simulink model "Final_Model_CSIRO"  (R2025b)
settings: Solver=ode23tb  StartTime=0.0  StopTime=50  RelTol=1e-3
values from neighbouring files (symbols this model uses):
  C_4 = 0.1670*C_b    (= 1.00487241952e-06)    [VSM_CSIRO.m]    (also in VSM.m)
  C_6 = 0.2835*C_b    (= 1.70587623314e-06)    [VSM_CSIRO.m]    (also in VSM.m)
  C_8 = 0.2275*C_b    (= 1.36891302659e-06)    [VSM_CSIRO.m]    (also in VSM.m)
  C_dc = 0.008*(n)    (= 1.6)    [VSM_CSIRO.m]    (also in VSM.m)
  C_f = n*300*10^-6    (= 0.06)    [VSM_CSIRO.m]    (also in VSM.m)
  D_p = (1/(m_p*w_b))    (= 101321.183642)    [VSM_CSIRO.m]    (also in VSM.m)
  droop_percentage = 1    [VSM_CSIRO.m]    (also in VSM.m = 5)
  i_ll = -1.15*(S_b/Vdc_n)-i_loss_dc    [VSM_CSIRO.m]    (also in VSM.m)
  i_ul = 1.15*(S_b/Vdc_n)+i_loss_dc    [VSM_CSIRO.m]    (also in VSM.m)
  J = D_p*tau_f    (= 2026.42367285)    [VSM_CSIRO.m]    (also in VSM.m)
  k_dc = eta_1/(Vdc_n*m_p)    [VSM_CSIRO.m]    (also in VSM.m)
  K_p = (1/Vdc_n)    [VSM_CSIRO.m]    (also in VSM.m)
  K_r = 1/R_dc    [VSM_CSIRO.m]    (also in VSM.m)
  Kff_i = 1    [VSM_CSIRO.m]    (also in VSM.m)
  Kff_v = 1    [VSM_CSIRO.m]    (also in VSM.m)
  Ki_i = (1/n)*1.19    (= 0.00595)    [VSM_CSIRO.m]    (also in VSM.m)
  Ki_v = (n)*1.161022    (= 232.2044)    [VSM_CSIRO.m]    (also in VSM.m)
  ki_v_ac = 4*5.2500e-04    (= 0.0021)    [VSM_CSIRO.m]    (also in VSM.m)
  Kp_i = 0.738891    [VSM_CSIRO.m]    (also in VSM.m)
  Kp_v = 0.52    [VSM_CSIRO.m]    (also in VSM.m)
  kp_v_ac = 0.001    [VSM_CSIRO.m]    (also in VSM.m)
  L1_pu = 1*0.0186/m    (= 0.000186)    [VSM_CSIRO.m]    (also in VSM.m)
  L_45 = L_lines(2)    [VSM_CSIRO.m]    (also in VSM.m)
  L_56 = L_lines(3)    [VSM_CSIRO.m]    (also in VSM.m)
  L_67 = L_lines(5)    [VSM_CSIRO.m]    (also in VSM.m)
  L_78 = L_lines(6)    [VSM_CSIRO.m]    (also in VSM.m)
  L_89 = L_lines(8)    [VSM_CSIRO.m]    (also in VSM.m)
  L_94 = L_lines(9)    [VSM_CSIRO.m]    (also in VSM.m)
  L_f = (1/n)*200*10^-6    (= 1e-06)    [VSM_CSIRO.m]    (also in VSM.m)
  n = 200    [VSM_CSIRO.m]    (also in VSM.m)
  pl = S_b*ps    (= 75000000)    [VSM_CSIRO.m]    (also in VSM.m)
  ps = base/3    (= 0.75)    [VSM_CSIRO.m]    (also in VSM.m)
  R1_pu = 1*0.00734/m    (= 7.34e-05)    [VSM_CSIRO.m]    (also in VSM.m)
  R_45 = R_lines(2)    [VSM_CSIRO.m]    (also in VSM.m)
  R_56 = R_lines(3)    [VSM_CSIRO.m]    (also in VSM.m)
  R_67 = R_lines(5)    [VSM_CSIRO.m]    (also in VSM.m)
  R_78 = R_lines(6)    [VSM_CSIRO.m]    (also in VSM.m)
  R_89 = R_lines(8)    [VSM_CSIRO.m]    (also in VSM.m)
  R_94 = R_lines(9)    [VSM_CSIRO.m]    (also in VSM.m)
  R_dc = (Vdc_n/(0.05*(S_b)/Vdc_n))    [VSM_CSIRO.m]    (also in VSM.m)
  R_f = 0.001/n    (= 5e-06)    [VSM_CSIRO.m]    (also in VSM.m)
  S_b = 100*(10^6)    (= 100000000)    [VSM_CSIRO.m]    (also in VSM.m)
  S_bt = S_b    (= 100000000)    [VSM_CSIRO.m]    (also in VSM.m)
  T_en = T_load-0.5    (= 44.5)    [VSM_CSIRO.m]    (also in VSM.m = 24.5)
  t_l = 2    [VSM_CSIRO.m]
  tau_dc = 0.05    [VSM_CSIRO.m]    (also in VSM.m)
  tau_g = 5    [VSM_CSIRO.m]    (also in VSM.m)
  V1_rms = 1000    [VSM_CSIRO.m]    (also in VSM.m)
  V2_rms = 13800    [VSM_CSIRO.m]    (also in VSM.m)
  V_m = sqrt(2/3)*V1_rms    [VSM_CSIRO.m]    (also in VSM.m)
  Vdc_n = 3*V_m    [VSM_CSIRO.m]    (also in VSM.m)
  w_b = 2*pi*f_b    (= 314.159265359)    [VSM_CSIRO.m]    (also in VSM.m)
  w_f = 2*pi*5    (= 31.4159265359)    [VSM_CSIRO.m]    (also in VSM.m)
undefined symbols (not defined in the file or in its folder): D1, Delta, DiscIntNeverNeededParam, i_dc
libraries: spsSeriesRLCBranchLib x142, spsThreePhaseVIMeasurementLib x69, slpidlib x44, spsabctodq0Lib x44, spsVoltageMeasurementLib x28, spsGroundLib x23, spsThreePhaseBreakerLib x23, spsThreePhaseParallelRLCLoadLib x21, spsdq0toabcLib x16, spsUniversalBridgeLib x16, spsPowerPositiveSequenceLib x14, spsDCVoltageSourceLib x14
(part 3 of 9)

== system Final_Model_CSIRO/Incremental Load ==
  Base Load {1..6,8..12} (11 alike) : spsThreePhaseParallelRLCLoadLib/Three-Phase Parallel RLC Load  LConnTagsString=A|B|C  Configuration=Y (grounded)  NominalVoltage=230e3  Vabc=[1e3 1e3 1e3]  Vabcp=[1e3 1e3 1e3]  NominalFrequency=50  UnbalancedPower=off  ActivePower=pl-pl+10.04e6  InductivePower=0  CapacitivePower=0  Pabc=[10e3 9e3 11e3]  QLabc=[100 90 110]  QCabc=[100 90 110]  Pabcp=[10e3 9e3 11e3]  QLabcp=[100 90 110]  QCabcp=[100 90 110]  Measurements=None  LoadType=constant Z
  Base Load {7,13..18} (7 alike) : spsThreePhaseParallelRLCLoadLib/Three-Phase Parallel RLC Load  LConnTagsString=A|B|C  Configuration=Y (grounded)  NominalVoltage=230e3  Vabc=[1e3 1e3 1e3]  Vabcp=[1e3 1e3 1e3]  NominalFrequency=50  UnbalancedPower=off  ActivePower=pl-pl+10e6  InductivePower=0  CapacitivePower=0  Pabc=[10e3 9e3 11e3]  QLabc=[100 90 110]  QCabc=[100 90 110]  Pabcp=[10e3 9e3 11e3]  QLabcp=[100 90 110]  QCabcp=[100 90 110]  Measurements=None  LoadType=constant Z
  Three-Phase Breaker1 : spsThreePhaseBreakerLib/Three-Phase Breaker  InitialState=open  SwitchA=on  SwitchB=on  SwitchC=on  SwitchTimes=10+2*t_l  External=off  BreakerResistance=0.01  SnubberResistance=1e6  SnubberCapacitance=inf  Measurements=None
  Three-Phase Breaker10 : spsThreePhaseBreakerLib/Three-Phase Breaker  InitialState=open  SwitchA=on  SwitchB=on  SwitchC=on  SwitchTimes=10+9*t_l  External=off  BreakerResistance=0.01  SnubberResistance=1e6  SnubberCapacitance=inf  Measurements=None
  Three-Phase Breaker11 : spsThreePhaseBreakerLib/Three-Phase Breaker  InitialState=open  SwitchA=on  SwitchB=on  SwitchC=on  SwitchTimes=10+10*t_l  External=off  BreakerResistance=0.01  SnubberResistance=1e6  SnubberCapacitance=inf  Measurements=None
  Three-Phase Breaker12 : spsThreePhaseBreakerLib/Three-Phase Breaker  InitialState=open  SwitchA=on  SwitchB=on  SwitchC=on  SwitchTimes=10+11*t_l  External=off  BreakerResistance=0.01  SnubberResistance=1e6  SnubberCapacitance=inf  Measurements=None
  Three-Phase Breaker13 : spsThreePhaseBreakerLib/Three-Phase Breaker  InitialState=open  SwitchA=on  SwitchB=on  SwitchC=on  SwitchTimes=10+15*t_l  External=off  BreakerResistance=0.01  SnubberResistance=1e6  SnubberCapacitance=inf  Measurements=None
  Three-Phase Breaker14 : spsThreePhaseBreakerLib/Three-Phase Breaker  InitialState=open  SwitchA=on  SwitchB=on  SwitchC=on  SwitchTimes=10+16*t_l  External=off  BreakerResistance=0.01  SnubberResistance=1e6  SnubberCapacitance=inf  Measurements=None
  Three-Phase Breaker15 : spsThreePhaseBreakerLib/Three-Phase Breaker  InitialState=open  SwitchA=on  SwitchB=on  SwitchC=on  SwitchTimes=10+17*t_l  External=off  BreakerResistance=0.01  SnubberResistance=1e6  SnubberCapacitance=inf  Measurements=None
  Three-Phase Breaker16 : spsThreePhaseBreakerLib/Three-Phase Breaker  InitialState=open  SwitchA=on  SwitchB=on  SwitchC=on  SwitchTimes=10+12*t_l  External=off  BreakerResistance=0.01  SnubberResistance=1e6  SnubberCapacitance=inf  Measurements=None
  Three-Phase Breaker17 : spsThreePhaseBreakerLib/Three-Phase Breaker  InitialState=open  SwitchA=on  SwitchB=on  SwitchC=on  SwitchTimes=10+13*t_l  External=off  BreakerResistance=0.01  SnubberResistance=1e6  SnubberCapacitance=inf  Measurements=None
  Three-Phase Breaker18 : spsThreePhaseBreakerLib/Three-Phase Breaker  InitialState=open  SwitchA=on  SwitchB=on  SwitchC=on  SwitchTimes=10+14*t_l  External=off  BreakerResistance=0.01  SnubberResistance=1e6  SnubberCapacitance=inf  Measurements=None
  Three-Phase Breaker2 : spsThreePhaseBreakerLib/Three-Phase Breaker  InitialState=open  SwitchA=on  SwitchB=on  SwitchC=on  SwitchTimes=10+t_l  External=off  BreakerResistance=0.01  SnubberResistance=1e6  SnubberCapacitance=inf  Measurements=None
  Three-Phase Breaker3 : spsThreePhaseBreakerLib/Three-Phase Breaker  InitialState=open  SwitchA=on  SwitchB=on  SwitchC=on  SwitchTimes=10  External=off  BreakerResistance=0.01  SnubberResistance=1e6  SnubberCapacitance=inf  Measurements=None
  Three-Phase Breaker4 : spsThreePhaseBreakerLib/Three-Phase Breaker  InitialState=open  SwitchA=on  SwitchB=on  SwitchC=on  SwitchTimes=10+3*t_l  External=off  BreakerResistance=0.01  SnubberResistance=1e6  SnubberCapacitance=inf  Measurements=None
  Three-Phase Breaker5 : spsThreePhaseBreakerLib/Three-Phase Breaker  InitialState=open  SwitchA=on  SwitchB=on  SwitchC=on  SwitchTimes=10+4*t_l  External=off  BreakerResistance=0.01  SnubberResistance=1e6  SnubberCapacitance=inf  Measurements=None
  Three-Phase Breaker6 : spsThreePhaseBreakerLib/Three-Phase Breaker  InitialState=open  SwitchA=on  SwitchB=on  SwitchC=on  SwitchTimes=10+5*t_l  External=off  BreakerResistance=0.01  SnubberResistance=1e6  SnubberCapacitance=inf  Measurements=None
  Three-Phase Breaker7 : spsThreePhaseBreakerLib/Three-Phase Breaker  InitialState=open  SwitchA=on  SwitchB=on  SwitchC=on  SwitchTimes=10+6*t_l  External=off  BreakerResistance=0.01  SnubberResistance=1e6  SnubberCapacitance=inf  Measurements=None
  Three-Phase Breaker8 : spsThreePhaseBreakerLib/Three-Phase Breaker  InitialState=open  SwitchA=on  SwitchB=on  SwitchC=on  SwitchTimes=10+7*t_l  External=off  BreakerResistance=0.01  SnubberResistance=1e6  SnubberCapacitance=inf  Measurements=None
  Three-Phase Breaker9 : spsThreePhaseBreakerLib/Three-Phase Breaker  InitialState=open  SwitchA=on  SwitchB=on  SwitchC=on  SwitchTimes=10+8*t_l  External=off  BreakerResistance=0.01  SnubberResistance=1e6  SnubberCapacitance=inf  Measurements=None
  C : PMIOPort  Side=Left
  B : PMIOPort  Port=2  Side=Left
  A : PMIOPort  Port=3  Side=Left
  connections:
  Three-Phase Breaker10/LConn2 -- Three-Phase Breaker11/LConn2 -- Three-Phase Breaker9/LConn2 -- Three-Phase Breaker8/LConn2 -- Three-Phase Breaker3/LConn2 -- B/RConn1 -- Three-Phase Breaker2/LConn2 -- Three-Phase Breaker1/LConn2 -- Three-Phase Breaker4/LConn2 -- Three-Phase Breaker5/LConn2 -- Three-Phase Breaker6/LConn2 -- Three-Phase Breaker7/LConn2
  Three-Phase Breaker2/RConn3 -- Base Load 1/LConn1
  Three-Phase Breaker10/LConn1 -- Three-Phase Breaker11/LConn1 -- Three-Phase Breaker9/LConn1 -- Three-Phase Breaker8/LConn1 -- Three-Phase Breaker7/LConn1 -- Three-Phase Breaker2/LConn1 -- A/RConn1 -- Three-Phase Breaker3/LConn1 -- Three-Phase Breaker1/LConn1 -- Three-Phase Breaker4/LConn1 -- Three-Phase Breaker5/LConn1 -- Three-Phase Breaker6/LConn1
  Three-Phase Breaker3/RConn1 -- Base Load 7/LConn3
  Three-Phase Breaker10/LConn3 -- Three-Phase Breaker11/LConn3 -- Three-Phase Breaker9/LConn3 -- Three-Phase Breaker8/LConn3 -- Three-Phase Breaker3/LConn3 -- C/RConn1 -- Three-Phase Breaker2/LConn3 -- Three-Phase Breaker1/LConn3 -- Three-Phase Breaker4/LConn3 -- Three-Phase Breaker5/LConn3 -- Three-Phase Breaker6/LConn3 -- Three-Phase Breaker7/LConn3
  Three-Phase Breaker2/RConn1 -- Base Load 1/LConn3
  Three-Phase Breaker3/RConn2 -- Base Load 7/LConn2
  Three-Phase Breaker3/RConn3 -- Base Load 7/LConn1
  Three-Phase Breaker2/RConn2 -- Base Load 1/LConn2
  Three-Phase Breaker1/RConn1 -- Base Load 2/LConn3
  Three-Phase Breaker1/RConn2 -- Base Load 2/LConn2
  Three-Phase Breaker4/RConn1 -- Base Load 3/LConn3
  Three-Phase Breaker4/RConn2 -- Base Load 3/LConn2
  Three-Phase Breaker5/RConn1 -- Base Load 4/LConn3
  Three-Phase Breaker5/RConn2 -- Base Load 4/LConn2
  Three-Phase Breaker1/RConn3 -- Base Load 2/LConn1
  Three-Phase Breaker4/RConn3 -- Base Load 3/LConn1
  Three-Phase Breaker6/RConn2 -- Base Load 5/LConn2
  Three-Phase Breaker6/RConn1 -- Base Load 5/LConn3
  Three-Phase Breaker5/RConn3 -- Base Load 4/LConn1
  Three-Phase Breaker6/RConn3 -- Base Load 5/LConn1
  Three-Phase Breaker7/RConn2 -- Base Load 6/LConn2
  Three-Phase Breaker7/RConn1 -- Base Load 6/LConn3
  Three-Phase Breaker7/RConn3 -- Base Load 6/LConn1
  Three-Phase Breaker8/RConn1 -- Base Load 8/LConn3
  Three-Phase Breaker9/RConn1 -- Base Load 9/LConn3
  Three-Phase Breaker9/RConn3 -- Base Load 9/LConn1
  Three-Phase Breaker11/RConn2 -- Base Load 11/LConn2
  Three-Phase Breaker10/RConn3 -- Base Load 10/LConn1
  Three-Phase Breaker11/RConn1 -- Base Load 11/LConn3
  Three-Phase Breaker8/RConn3 -- Base Load 8/LConn1
  Three-Phase Breaker11/RConn3 -- Base Load 11/LConn1
  Three-Phase Breaker10/RConn2 -- Base Load 10/LConn2
  Three-Phase Breaker12/RConn1 -- Base Load 12/LConn3
  Three-Phase Breaker8/RConn2 -- Base Load 8/LConn2
  Three-Phase Breaker10/RConn1 -- Base Load 10/LConn3
  Three-Phase Breaker12/RConn2 -- Base Load 12/LConn2
  Three-Phase Breaker9/RConn2 -- Base Load 9/LConn2
  Three-Phase Breaker14/RConn3 -- Base Load 14/LConn1
  Three-Phase Breaker16/RConn2 -- Base Load 16/LConn2
  Three-Phase Breaker16/RConn3 -- Base Load 16/LConn1
  Three-Phase Breaker17/RConn3 -- Base Load 17/LConn1
  Three-Phase Breaker17/RConn2 -- Base Load 17/LConn2
  Three-Phase Breaker13/RConn2 -- Base Load 13/LConn2
  Three-Phase Breaker15/RConn2 -- Base Load 15/LConn2
  Three-Phase Breaker13/RConn3 -- Base Load 13/LConn1
  Three-Phase Breaker18/RConn2 -- Base Load 18/LConn2
  Three-Phase Breaker18/RConn1 -- Base Load 18/LConn3
  Three-Phase Breaker14/RConn1 -- Base Load 14/LConn3
  Three-Phase Breaker14/RConn2 -- Base Load 14/LConn2
  Three-Phase Breaker17/RConn1 -- Base Load 17/LConn3
  Three-Phase Breaker15/RConn1 -- Base Load 15/LConn3
  Three-Phase Breaker15/RConn3 -- Base Load 15/LConn1
  Three-Phase Breaker18/RConn3 -- Base Load 18/LConn1
  Three-Phase Breaker13/RConn1 -- Base Load 13/LConn3
  Three-Phase Breaker16/RConn1 -- Base Load 16/LConn3
  Three-Phase Breaker18/LConn2 -- Three-Phase Breaker15/LConn2 -- Three-Phase Breaker14/LConn2 -- Three-Phase Breaker13/LConn2
  Three-Phase Breaker15/LConn1 -- Three-Phase Breaker14/LConn1 -- Three-Phase Breaker18/LConn1 -- Three-Phase Breaker13/LConn1
  Three-Phase Breaker15/LConn3 -- Three-Phase Breaker14/LConn3 -- Three-Phase Breaker18/LConn3 -- Three-Phase Breaker13/LConn3
  Base Load 12/LConn1 -- Three-Phase Breaker12/RConn3
  Three-Phase Breaker12/LConn2 -- Three-Phase Breaker16/LConn2
  Three-Phase Breaker12/LConn1 -- Three-Phase Breaker16/LConn1
  Three-Phase Breaker12/LConn3 -- Three-Phase Breaker16/LConn3

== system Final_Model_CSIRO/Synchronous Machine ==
  Pset : Inport
  Bus Selector3 : BusSelector  OutputSignals="dq0 components.Stator voltage  vq (pu),dq0 components.Stator voltage  vd (pu),Output active power   Peo (pu),Output reactive power  Qeo (pu),Mechanical.Rotor mechanical angle  theta (deg),Mechanical.Rotor speed deviation  dw (pu),dq0 components.Field current  ifd (pu),Mechanical.Rotor speed  wm (pu)"
  Gain : Gain  Gain=50
  Generic Power System Stabilizer : spsGenericPowerSystemStabilizerLib/Generic Power System Stabilizer  Tsensor=30e-4  K=2.5  Twashout=2  Tleadlag1=[2*50e-3 0.01*20e-3]  Tleadlag2=[2*3 0.1*5.4]  VSlimits=2*[-0.15 0.15]  Vinit=0  Plot_On=off  MagdB_On=on  FreqRange=logspace(-2,2,500)
  LTI System3 : cstblocks/LTI System  sys=tf(1,[tau_g 1])  IC=[]  PadeOrder=0
  Mux1 : Mux  Inputs=2
  Mux3 : Mux  Inputs=2
  Positive Sequence Voltage1 : Fcn  Expr=sqrt(u(1)^2 + u(2)^2)
  Positive Sequence Voltage2 : Fcn  Expr=sqrt(u(1)^2 + u(2)^2)
  ST1A Excitation System : spsST1AExcitationSystemLib/ST1A Excitation System  Tr=20e-4  KaTa=[210 0.001]  VIminmax=[-999 +999]  VAminmax=[-999 999]  VRminmax=[-6.0 6.43]  KfTf=[0.001 1]  TbTc=[0 0 0 0]  KLR=1  ILR=2  Kc=0.038  v0=[1 1]  TsBlock=0
  Subsystem2 : Subsystem
  Synchronous Machine pu Fundamental : spsSynchronousMachinepuFundamentalLib/Synchronous Machine pu Fundamental  PresetModel=No  MechanicalLoad=Mechanical power Pm  ShowDetailedParameters=on  RotorType=Salient-pole  Units=per unit fundamental parameters  MeasurementBus=off  NominalParameters="[100E6  V2_rms   50]"  Stator="[ 2.85E-03  0.114  1.19  0.36 ]"  Field="[ 5.79E-04  0.114]"  Dampers2=[0.0652, 0.5134, 0.0287, 0.2553, 7.765e-3, 0.9167 ]  Dampers1="[ 1.17E-02  0.182  1.97E-02  0.384 ]"  Mechanical=[ 3.7 0 20]  PolePairs=20  InitialConditions="[ 0  0  0  0  0  0  0  0  1 ]"  SetSaturation=off  Saturation=[0.6404,0.7127,0.8441,0.9214,0.9956,1.082,1.19,1.316,1.457;0.7,0.7698,0.8872,0.9466,0.9969,1.046,1.1,1.151,1.201]  LoadFlowParameters=[1,0,0,0,0]  TsPowergui=0  TsBlock=-1  IterativeModel=Trapezoidal non iterative  IterativeDiscreteModel=Trapezoidal non iterative  BusType=PV  Pref=0  Qref=0  Qmin=-inf  Qmax=inf  PLF=0  QLF=0
  Terminal Load : spsThreePhaseParallelRLCLoadLib/Three-Phase Parallel RLC Load  LConnTagsString=A|B|C  Configuration=Y (grounded)  NominalVoltage=V2_rms  Vabc=[1e3 1e3 1e3]  Vabcp=[1e3 1e3 1e3]  NominalFrequency=50  UnbalancedPower=off  ActivePower=1  InductivePower=0  CapacitivePower=0  Pabc=[10e3 9e3 11e3]  QLabc=[100 90 110]  QCabc=[100 90 110]  Pabcp=[10e3 9e3 11e3]  QLabcp=[100 90 110]  QCabcp=[100 90 110]  Measurements=None  LoadType=constant Z
  wref6 : Constant
  wref7 : Constant
  A : PMIOPort  Side=Right
  B : PMIOPort  Port=2  Side=Right
  C : PMIOPort  Port=3  Side=Right
  f : Outport  VectorParamsAs1DForOutWhenUnconnected=off
  V : Outport  Port=2  VectorParamsAs1DForOutWhenUnconnected=off
  P : Outport  Port=3  VectorParamsAs1DForOutWhenUnconnected=off
  Theta : Outport  Port=4  VectorParamsAs1DForOutWhenUnconnected=off
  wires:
  Gain/1 -> f/1
  Pset/1 -> Subsystem2/1(P_ref)
  Positive Sequence Voltage2/1 -> V/1
  wref7/1 -> Subsystem2/2(speed_ref)
  wref6/1 -> ST1A Excitation System/1
  Mux3/1 -> Positive Sequence Voltage2/1
  Synchronous Machine pu Fundamental/1 -> Bus Selector3/1
  [w] -> Gain/1
  [Vq] -> Mux3/1
  [Vd] -> Mux3/2
  [P] -> P/1
  [Theta] -> Theta/1
  [w] -> Subsystem2/3(speed)
  Subsystem2/1(throttle) -> LTI System3/1
  Bus Selector3/1 -> [Vq]  "<Stator voltage  vq (pu)>"
  Bus Selector3/2 -> [Vd]  "<Stator voltage  vd (pu)>"
  Bus Selector3/3 -> [P]  "<Output active power   Peo (pu)>"
  Bus Selector3/4 -> [Q]  "<Output reactive power  Qeo (pu)>"
  Bus Selector3/5 -> [Theta]  "<Rotor mechanical angle  theta (deg)>"
  Bus Selector3/6 -> [dw]  "<Rotor speed deviation  dw (pu)>"
  Bus Selector3/7 -> [Ifd]  "<Field current  ifd (pu)>"
  Bus Selector3/8 -> [w]  "<Rotor speed  wm (pu)>"
  LTI System3/1 -> Synchronous Machine pu Fundamental/1
  Generic Power System Stabilizer/1 -> ST1A Excitation System/4
  [dw] -> Generic Power System Stabilizer/1
  [Ifd] -> ST1A Excitation System/3
  Mux1/1 -> Positive Sequence Voltage1/1
  [Vd] -> Mux1/1
  [Vq] -> Mux1/2
  Positive Sequence Voltage1/1 -> ST1A Excitation System/2
  ST1A Excitation System/1 -> Synchronous Machine pu Fundamental/2
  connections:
  Terminal Load/LConn1 -- Synchronous Machine pu Fundamental/RConn1 -- A/RConn1
  Terminal Load/LConn3 -- Synchronous Machine pu Fundamental/RConn3 -- C/RConn1
  Terminal Load/LConn2 -- Synchronous Machine pu Fundamental/RConn2 -- B/RConn1

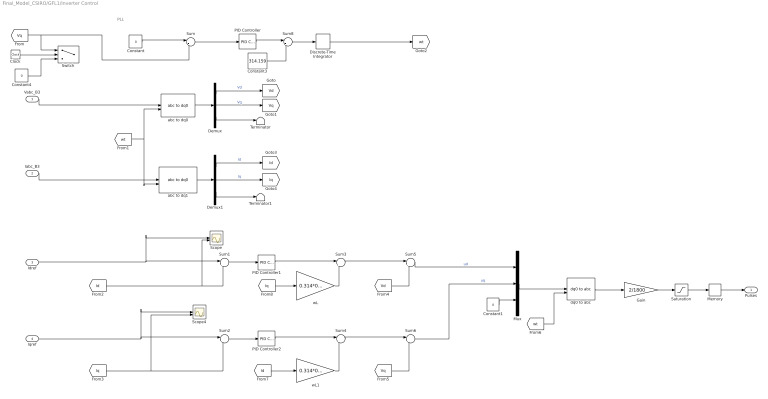
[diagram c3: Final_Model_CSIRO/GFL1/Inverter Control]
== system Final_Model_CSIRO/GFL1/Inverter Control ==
  note: PLL
  Vabc_B3 : Inport
  Iabc_B3 : Inport  Port=2
  Idref : Inport  Port=3
  Iqref : Inport  Port=4
  Clock : Clock
  Constant : Constant  Value=0  SampleTime=-1
  Constant1 : Constant  Value=0  SampleTime=-1
  Constant3 : Constant  Value=314.159  SampleTime=-1
  Constant4 : Constant  Value=0
  Demux : Demux  Outputs=3
  Demux1 : Demux  Outputs=3
  Discrete-Time Integrator : DiscreteIntegrator  SampleTime=-1  ICPrevOutput=DiscIntNeverNeededParam  ICPrevScaledInput=DiscIntNeverNeededParam
  Gain : Gain  Gain=2/1800
  Memory : Memory
  Mux : Mux  Inputs=3
  PID Controller : slpidlib/PID Controller  Controller=PI  Form=Parallel  TimeDomain=Discrete-time  UseExternalTs=off  SampleTime=-1  IntegratorMethod=Forward Euler  FilterMethod=Forward Euler  ControllerParametersSource=internal  P=0.02  I=50  UseKiTs=off  D=0  UseExternalDerivativeSource=off  N=100  UseFilter=on  TunerSelectOption=Transfer Function Based (PID Tuner App)  InitialConditionSource=internal  InitialConditionForIntegrator=0  InitialConditionForFilter=0  DifferentiatorICPrevScaledInput=0  ExternalReset=none  TrackingMode=off  Kt=1  LimitOutput=off  SatLimitsSource=internal  UpperSaturationLimit=inf  LowerSaturationLimit=-inf  LinearizeAsGain=on  AntiWindupMode=none  Kb=1  LimitIntegrator=off  UpperIntegratorSaturationLimit=inf  LowerIntegratorSaturationLimit=-inf  POutMin=[]  POutMax=[]  IOutMin=[]  IOutMax=[]  DOutMin=[]  DOutMax=[]  NOutMin=[]  NOutMax=[]  SumOutMin=[]  SumOutMax=[]  SaturationOutMin=[]  SaturationOutMax=[]  PParamMin=[]  PParamMax=[]  IParamMin=[]  IParamMax=[]  DParamMin=[]  DParamMax=[]  NParamMin=[]  NParamMax=[]  KbParamMin=[]  KbParamMax=[]  KtParamMin=[]  KtParamMax=[]  KbOutMin=[]  KbOutMax=[]  KtOutMin=[]  KtOutMax=[]  IntegratorOutMin=[]  IntegratorOutMax=[]  FilterOutMin=[]  FilterOutMax=[]  SumI1OutMin=[]  SumI1OutMax=[]  SumI2OutMin=[]  SumI2OutMax=[]  SumI3OutMin=[]  SumI3OutMax=[]  SumI4OutMin=[]  SumI4OutMax=[]  SumDOutMin=[]  SumDOutMax=[]  DifferentiatorOutMin=[]  DifferentiatorOutMax=[]  FilterDiffOutCoefMin=[]  FilterDiffOutCoefMax=[]  ReciprocalOutMin=[]  ReciprocalOutMax=[]  SumDenOutMin=[]  SumDenOutMax=[]  SumNumOutMin=[]  SumNumOutMax=[]  DivideOutMin=[]  DivideOutMax=[]  UdiffTsProdOutMin=[]  UdiffTsProdOutMax=[]  NTsProdOutMin=[]  NTsProdOutMax=[]  UintegralTsProdOutMin=[]  UintegralTsProdOutMax=[]  UngainTsProdOutMin=[]  UngainTsProdOutMax=[]  ClampingZeroOutDataTypeStr=Inherit: Inherit via back propagation  ClampingZeroOutMin=[]  ClampingZeroOutMax=[]  FilterDenConstantOutDataTypeStr=Inherit: Inherit via back propagation  FilterDenConstantOutMin=[]  FilterDenConstantOutMax=[]  PCopyOutDataTypeStr=Inherit: Inherit via back propagation  PCopyOutMin=[]  PCopyOutMax=[]  NCopyOutDataTypeStr=Inherit: Inherit via back propagation  NCopyOutMin=[]  NCopyOutMax=[]  IntegratorContinuousStateAttributes=''  IntegratorStateMustResolveToSignalObject=off  IntegratorRTWStateStorageClass=Auto  FilterContinuousStateAttributes=''  FilterStateMustResolveToSignalObject=off  FilterRTWStateStorageClass=Auto  ParallelPVariant=InternalParameters  IdealPVariant=Disabled  IVariant=InternalParameters  DVariant=Disabled  IntegratorVariant=Discrete  SatVariant=Disabled  AWVariant=Passthrough  PCopyVariant=Disabled  TRVariant=Disabled  FdbkBlocksVariant=Forward  IdealPFdbkVariant=Disabled  SatFdbkVariant=Disabled  DerivativeFilterVariant=Disabled  NVariant=Disabled  NCopyVariant=Disabled_SignalSpec  FilterICVariant=Disabled  IntegratorICVariant=InternalICs  ExternalResetVariant=Disabled  TRSumVariant=Passthrough  SumFdbkVariant=Disabled  SumVariant=Sum_PI  TsampFilterVariant=InternalTs  TsampNgainVariant=Passthrough  TsampIntegralVariant=Disabled_SignalSpec  ExternalSaturationOutDataTypeStr=Inherit: Same as second input  DerivativeSourceVariant=Disabled  PreIntVariant=InternalPreInt
  PID Controller1 : slpidlib/PID Controller  Controller=PI  Form=Parallel  TimeDomain=Discrete-time  UseExternalTs=off  SampleTime=-1  IntegratorMethod=Forward Euler  FilterMethod=Forward Euler  ControllerParametersSource=internal  P=0.1  I=10000/200  UseKiTs=off  D=0  UseExternalDerivativeSource=off  N=100  UseFilter=on  TunerSelectOption=Transfer Function Based (PID Tuner App)  InitialConditionSource=internal  InitialConditionForIntegrator=0  InitialConditionForFilter=0  DifferentiatorICPrevScaledInput=0  ExternalReset=none  TrackingMode=off  Kt=1  LimitOutput=on  SatLimitsSource=internal  UpperSaturationLimit=20e3  LowerSaturationLimit=-20e3  LinearizeAsGain=on  AntiWindupMode=none  Kb=1  LimitIntegrator=off  UpperIntegratorSaturationLimit=inf  LowerIntegratorSaturationLimit=-inf  POutMin=[]  POutMax=[]  IOutMin=[]  IOutMax=[]  DOutMin=[]  DOutMax=[]  NOutMin=[]  NOutMax=[]  SumOutMin=[]  SumOutMax=[]  SaturationOutMin=[]  SaturationOutMax=[]  PParamMin=[]  PParamMax=[]  IParamMin=[]  IParamMax=[]  DParamMin=[]  DParamMax=[]  NParamMin=[]  NParamMax=[]  KbParamMin=[]  KbParamMax=[]  KtParamMin=[]  KtParamMax=[]  KbOutMin=[]  KbOutMax=[]  KtOutMin=[]  KtOutMax=[]  IntegratorOutMin=[]  IntegratorOutMax=[]  FilterOutMin=[]  FilterOutMax=[]  SumI1OutMin=[]  SumI1OutMax=[]  SumI2OutMin=[]  SumI2OutMax=[]  SumI3OutMin=[]  SumI3OutMax=[]  SumI4OutMin=[]  SumI4OutMax=[]  SumDOutMin=[]  SumDOutMax=[]  DifferentiatorOutMin=[]  DifferentiatorOutMax=[]  FilterDiffOutCoefMin=[]  FilterDiffOutCoefMax=[]  ReciprocalOutMin=[]  ReciprocalOutMax=[]  SumDenOutMin=[]  SumDenOutMax=[]  SumNumOutMin=[]  SumNumOutMax=[]  DivideOutMin=[]  DivideOutMax=[]  UdiffTsProdOutMin=[]  UdiffTsProdOutMax=[]  NTsProdOutMin=[]  NTsProdOutMax=[]  UintegralTsProdOutMin=[]  UintegralTsProdOutMax=[]  UngainTsProdOutMin=[]  UngainTsProdOutMax=[]  ClampingZeroOutDataTypeStr=Inherit: Inherit via back propagation  ClampingZeroOutMin=[]  ClampingZeroOutMax=[]  FilterDenConstantOutDataTypeStr=Inherit: Inherit via back propagation  FilterDenConstantOutMin=[]  FilterDenConstantOutMax=[]  PCopyOutDataTypeStr=Inherit: Inherit via back propagation  PCopyOutMin=[]  PCopyOutMax=[]  NCopyOutDataTypeStr=Inherit: Inherit via back propagation  NCopyOutMin=[]  NCopyOutMax=[]  IntegratorContinuousStateAttributes=''  IntegratorStateMustResolveToSignalObject=off  IntegratorRTWStateStorageClass=Auto  FilterContinuousStateAttributes=''  FilterStateMustResolveToSignalObject=off  FilterRTWStateStorageClass=Auto  ParallelPVariant=InternalParameters  IdealPVariant=Disabled  IVariant=InternalParameters  DVariant=Disabled  IntegratorVariant=Discrete  SatVariant=Enabled  AWVariant=Passthrough  PCopyVariant=Disabled  TRVariant=Disabled  FdbkBlocksVariant=Forward  IdealPFdbkVariant=Disabled  SatFdbkVariant=Disabled  DerivativeFilterVariant=Disabled  NVariant=Disabled  NCopyVariant=Disabled_SignalSpec  FilterICVariant=Disabled  IntegratorICVariant=InternalICs  ExternalResetVariant=Disabled  TRSumVariant=Passthrough  SumFdbkVariant=Disabled  SumVariant=Sum_PI  TsampFilterVariant=InternalTs  TsampNgainVariant=Passthrough  TsampIntegralVariant=Disabled_SignalSpec  ExternalSaturationOutDataTypeStr=Inherit: Same as second input  DerivativeSourceVariant=Disabled  PreIntVariant=InternalPreInt
  PID Controller2 : slpidlib/PID Controller  Controller=PI  Form=Parallel  TimeDomain=Discrete-time  UseExternalTs=off  SampleTime=-1  IntegratorMethod=Forward Euler  FilterMethod=Forward Euler  ControllerParametersSource=internal  P=0.1  I=1000/2  UseKiTs=off  D=0  UseExternalDerivativeSource=off  N=100  UseFilter=on  TunerSelectOption=Transfer Function Based (PID Tuner App)  InitialConditionSource=internal  InitialConditionForIntegrator=0  InitialConditionForFilter=0  DifferentiatorICPrevScaledInput=0  ExternalReset=none  TrackingMode=off  Kt=1  LimitOutput=on  SatLimitsSource=internal  UpperSaturationLimit=20e3  LowerSaturationLimit=-20e3  LinearizeAsGain=on  AntiWindupMode=none  Kb=1  LimitIntegrator=off  UpperIntegratorSaturationLimit=inf  LowerIntegratorSaturationLimit=-inf  POutMin=[]  POutMax=[]  IOutMin=[]  IOutMax=[]  DOutMin=[]  DOutMax=[]  NOutMin=[]  NOutMax=[]  SumOutMin=[]  SumOutMax=[]  SaturationOutMin=[]  SaturationOutMax=[]  PParamMin=[]  PParamMax=[]  IParamMin=[]  IParamMax=[]  DParamMin=[]  DParamMax=[]  NParamMin=[]  NParamMax=[]  KbParamMin=[]  KbParamMax=[]  KtParamMin=[]  KtParamMax=[]  KbOutMin=[]  KbOutMax=[]  KtOutMin=[]  KtOutMax=[]  IntegratorOutMin=[]  IntegratorOutMax=[]  FilterOutMin=[]  FilterOutMax=[]  SumI1OutMin=[]  SumI1OutMax=[]  SumI2OutMin=[]  SumI2OutMax=[]  SumI3OutMin=[]  SumI3OutMax=[]  SumI4OutMin=[]  SumI4OutMax=[]  SumDOutMin=[]  SumDOutMax=[]  DifferentiatorOutMin=[]  DifferentiatorOutMax=[]  FilterDiffOutCoefMin=[]  FilterDiffOutCoefMax=[]  ReciprocalOutMin=[]  ReciprocalOutMax=[]  SumDenOutMin=[]  SumDenOutMax=[]  SumNumOutMin=[]  SumNumOutMax=[]  DivideOutMin=[]  DivideOutMax=[]  UdiffTsProdOutMin=[]  UdiffTsProdOutMax=[]  NTsProdOutMin=[]  NTsProdOutMax=[]  UintegralTsProdOutMin=[]  UintegralTsProdOutMax=[]  UngainTsProdOutMin=[]  UngainTsProdOutMax=[]  ClampingZeroOutDataTypeStr=Inherit: Inherit via back propagation  ClampingZeroOutMin=[]  ClampingZeroOutMax=[]  FilterDenConstantOutDataTypeStr=Inherit: Inherit via back propagation  FilterDenConstantOutMin=[]  FilterDenConstantOutMax=[]  PCopyOutDataTypeStr=Inherit: Inherit via back propagation  PCopyOutMin=[]  PCopyOutMax=[]  NCopyOutDataTypeStr=Inherit: Inherit via back propagation  NCopyOutMin=[]  NCopyOutMax=[]  IntegratorContinuousStateAttributes=''  IntegratorStateMustResolveToSignalObject=off  IntegratorRTWStateStorageClass=Auto  FilterContinuousStateAttributes=''  FilterStateMustResolveToSignalObject=off  FilterRTWStateStorageClass=Auto  ParallelPVariant=InternalParameters  IdealPVariant=Disabled  IVariant=InternalParameters  DVariant=Disabled  IntegratorVariant=Discrete  SatVariant=Enabled  AWVariant=Passthrough  PCopyVariant=Disabled  TRVariant=Disabled  FdbkBlocksVariant=Forward  IdealPFdbkVariant=Disabled  SatFdbkVariant=Disabled  DerivativeFilterVariant=Disabled  NVariant=Disabled  NCopyVariant=Disabled_SignalSpec  FilterICVariant=Disabled  IntegratorICVariant=InternalICs  ExternalResetVariant=Disabled  TRSumVariant=Passthrough  SumFdbkVariant=Disabled  SumVariant=Sum_PI  TsampFilterVariant=InternalTs  TsampNgainVariant=Passthrough  TsampIntegralVariant=Disabled_SignalSpec  ExternalSaturationOutDataTypeStr=Inherit: Same as second input  DerivativeSourceVariant=Disabled  PreIntVariant=InternalPreInt
  Saturation : Saturate  UpperLimit=1  LowerLimit=-1
  Scope : Scope  NumInputPorts=2
  Scope4 : Scope  NumInputPorts=2
  Sum : Sum  Inputs=|-+
  Sum1 : Sum  Inputs=|+-
  Sum2 : Sum  Inputs=|+-
  Sum3 : Sum  Inputs=|+-
  Sum{4..6,8} (4 alike) : Sum  Inputs=|++
  Switch : Switch  Criteria=u2 > Threshold  Threshold=10
  Terminator : Terminator
  Terminator1 : Terminator
  abc to dq0 : spsabctodq0Lib/abc to dq0  Alignment=90 degrees behind phase A axis
  abc to dq1 : spsabctodq0Lib/abc to dq0  Alignment=90 degrees behind phase A axis
  dq0 to abc : spsdq0toabcLib/dq0 to abc  Alignment=90 degrees behind phase A axis
  wL : Gain  Gain=0.314*0.003
  wL1 : Gain  Gain=0.314*0.003
  Pulses : Outport
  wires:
  abc to dq0/1 -> Demux/1
  Demux/3 -> Terminator/1
  Demux1/3 -> Terminator1/1
  abc to dq1/1 -> Demux1/1
  Iabc_B3/1 -> abc to dq1/1
  Constant/1 -> Sum/1
  Demux/2 -> [Vq]  "Vq"
  Sum/1 -> PID Controller/1
  PID Controller/1 -> Sum8/1
  [wt] -> abc to dq1/2, abc to dq0/2
  Demux1/1 -> [Id]  "Id"
  Demux1/2 -> [Iq]  "Iq"
  [Id] -> Scope/2, Sum1/2
  Iqref/1 -> Scope4/1, Sum2/1
  [Iq] -> Sum2/2, Scope4/2
  Sum1/1 -> PID Controller1/1
  Sum2/1 -> PID Controller2/1
  PID Controller1/1 -> Sum3/1
  PID Controller2/1 -> Sum4/1
  wL1/1 -> Sum4/2
  wL/1 -> Sum3/2
  Sum3/1 -> Sum5/1
  [Vd] -> Sum5/2
  Sum4/1 -> Sum6/1
  [Vq] -> Sum6/2
  Mux/1 -> dq0 to abc/1
  Sum5/1 -> Mux/1  "ud"
  Sum6/1 -> Mux/2  "uq"
  Constant1/1 -> Mux/3
  dq0 to abc/1 -> Gain/1
  Vabc_B3/1 -> abc to dq0/1
  Idref/1 -> Scope/1, Sum1/1
  [Id] -> wL1/1
  [Iq] -> wL/1
  Demux/1 -> [Vd]  "Vd"
  Gain/1 -> Saturation/1
  Memory/1 -> Pulses/1
  Discrete-Time Integrator/1 -> [wt]
  Saturation/1 -> Memory/1
  Constant3/1 -> Sum8/2
  Constant4/1 -> Switch/3
  Clock/1 -> Switch/2
  [Vq] -> Sum/2, Switch/1
  [wt] -> dq0 to abc/2
  Sum8/1 -> Discrete-Time Integrator/1

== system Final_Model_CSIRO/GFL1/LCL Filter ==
  Cf : spsSeriesRLCBranchLib/Series RLC Branch  LConnTagsString=__new0  RConnTagsString=__new0  BranchType=RC  Resistance=200  Inductance=0.0058  SetiL0=off  InitialCurrent=0  Capacitance=50e-6  Setx0=off  InitialVoltage=0  Measurements=None
  Cf1 : spsSeriesRLCBranchLib/Series RLC Branch  LConnTagsString=__new0  RConnTagsString=__new0  BranchType=RC  Resistance=200  Inductance=0.0058  SetiL0=off  InitialCurrent=0  Capacitance=50e-6  Setx0=off  InitialVoltage=0  Measurements=None
  Cf2 : spsSeriesRLCBranchLib/Series RLC Branch  LConnTagsString=__new0  RConnTagsString=__new0  BranchType=RC  Resistance=200  Inductance=0.0058  SetiL0=off  InitialCurrent=0  Capacitance=50e-6  Setx0=off  InitialVoltage=0  Measurements=None
  Ground : spsGroundLib/Ground  LConnTagsString=a
  Lg : spsSeriesRLCBranchLib/Series RLC Branch  LConnTagsString=__new0  RConnTagsString=__new0  BranchType=L  Resistance=0.2  Inductance=5e-6  SetiL0=off  InitialCurrent=0  Capacitance=1e-6  Setx0=off  InitialVoltage=0  Measurements=None
  Linv : spsSeriesRLCBranchLib/Series RLC Branch  LConnTagsString=__new0  RConnTagsString=__new0  BranchType=RL  Resistance=1e-3  Inductance=0.003e-3  SetiL0=off  InitialCurrent=0  Capacitance=1e-6  Setx0=off  InitialVoltage=0  Measurements=None
  Series RLC Branch1 : spsSeriesRLCBranchLib/Series RLC Branch  LConnTagsString=__new0  RConnTagsString=__new0  BranchType=RL  Resistance=1e-3  Inductance=0.003e-3  SetiL0=off  InitialCurrent=0  Capacitance=1e-6  Setx0=off  InitialVoltage=0  Measurements=None
  Series RLC Branch2 : spsSeriesRLCBranchLib/Series RLC Branch  LConnTagsString=__new0  RConnTagsString=__new0  BranchType=RL  Resistance=1e-3  Inductance=0.003e-3  SetiL0=off  InitialCurrent=0  Capacitance=1e-6  Setx0=off  InitialVoltage=0  Measurements=None
  Series RLC Branch3 : spsSeriesRLCBranchLib/Series RLC Branch  LConnTagsString=__new0  RConnTagsString=__new0  BranchType=L  Resistance=0.2  Inductance=5e-6  SetiL0=off  InitialCurrent=0  Capacitance=1e-6  Setx0=off  InitialVoltage=0  Measurements=None
  Series RLC Branch4 : spsSeriesRLCBranchLib/Series RLC Branch  LConnTagsString=__new0  RConnTagsString=__new0  BranchType=L  Resistance=0.2  Inductance=5e-6  SetiL0=off  InitialCurrent=0  Capacitance=1e-6  Setx0=off  InitialVoltage=0  Measurements=None
  Three-Phase V-I Measurement : spsThreePhaseVIMeasurementLib/Three-Phase V-I Measurement  VoltageMeasurement=phase-to-phase  SetLabelV=on  LabelV=Vabc_B2_2  Vpu=off  VpuLL=off  CurrentMeasurement=no  SetLabelI=off  LabelI=Iabc  Ipu=off  Pbase=100e6  Vbase=500e3  OutputType=Complex  PhasorSimulation=off  PSBequivalent=0
  A : PMIOPort  Side=Left
  a : PMIOPort  Port=2  Side=Right
  B : PMIOPort  Port=3  Side=Left
  b : PMIOPort  Port=4  Side=Right
  C : PMIOPort  Port=5  Side=Left
  c : PMIOPort  Port=6  Side=Right
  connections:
  A/RConn1 -- Linv/LConn1
  B/RConn1 -- Series RLC Branch1/LConn1
  C/RConn1 -- Series RLC Branch2/LConn1
  Lg/LConn1 -- Three-Phase V-I Measurement/LConn1 -- Linv/RConn1
  Series RLC Branch4/LConn1 -- Three-Phase V-I Measurement/LConn3 -- Series RLC Branch2/RConn1
  Series RLC Branch3/LConn1 -- Three-Phase V-I Measurement/LConn2 -- Series RLC Branch1/RConn1
  Cf1/LConn1 -- Ground/LConn1 -- Cf/LConn1 -- Cf2/LConn1
  Cf/RConn1 -- Three-Phase V-I Measurement/RConn1
  Cf1/RConn1 -- Three-Phase V-I Measurement/RConn2
  Cf2/RConn1 -- Three-Phase V-I Measurement/RConn3
  Lg/RConn1 -- a/RConn1
  Series RLC Branch3/RConn1 -- b/RConn1
  Series RLC Branch4/RConn1 -- c/RConn1

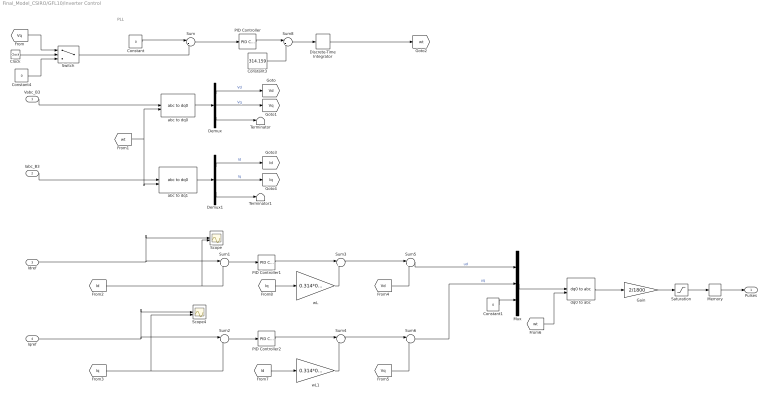
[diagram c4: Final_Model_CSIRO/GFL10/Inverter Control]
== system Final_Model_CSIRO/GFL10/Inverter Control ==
  note: PLL
  Vabc_B3 : Inport
  Iabc_B3 : Inport  Port=2
  Idref : Inport  Port=3
  Iqref : Inport  Port=4
  Clock : Clock
  Constant : Constant  Value=0  SampleTime=-1
  Constant1 : Constant  Value=0  SampleTime=-1
  Constant3 : Constant  Value=314.159  SampleTime=-1
  Constant4 : Constant  Value=0
  Demux : Demux  Outputs=3
  Demux1 : Demux  Outputs=3
  Discrete-Time Integrator : DiscreteIntegrator  SampleTime=-1  ICPrevOutput=DiscIntNeverNeededParam  ICPrevScaledInput=DiscIntNeverNeededParam
  Gain : Gain  Gain=2/1800
  Memory : Memory
  Mux : Mux  Inputs=3
  PID Controller : slpidlib/PID Controller  Controller=PI  Form=Parallel  TimeDomain=Discrete-time  UseExternalTs=off  SampleTime=-1  IntegratorMethod=Forward Euler  FilterMethod=Forward Euler  ControllerParametersSource=internal  P=0.02  I=50  UseKiTs=off  D=0  UseExternalDerivativeSource=off  N=100  UseFilter=on  TunerSelectOption=Transfer Function Based (PID Tuner App)  InitialConditionSource=internal  InitialConditionForIntegrator=0  InitialConditionForFilter=0  DifferentiatorICPrevScaledInput=0  ExternalReset=none  TrackingMode=off  Kt=1  LimitOutput=off  SatLimitsSource=internal  UpperSaturationLimit=inf  LowerSaturationLimit=-inf  LinearizeAsGain=on  AntiWindupMode=none  Kb=1  LimitIntegrator=off  UpperIntegratorSaturationLimit=inf  LowerIntegratorSaturationLimit=-inf  POutMin=[]  POutMax=[]  IOutMin=[]  IOutMax=[]  DOutMin=[]  DOutMax=[]  NOutMin=[]  NOutMax=[]  SumOutMin=[]  SumOutMax=[]  SaturationOutMin=[]  SaturationOutMax=[]  PParamMin=[]  PParamMax=[]  IParamMin=[]  IParamMax=[]  DParamMin=[]  DParamMax=[]  NParamMin=[]  NParamMax=[]  KbParamMin=[]  KbParamMax=[]  KtParamMin=[]  KtParamMax=[]  KbOutMin=[]  KbOutMax=[]  KtOutMin=[]  KtOutMax=[]  IntegratorOutMin=[]  IntegratorOutMax=[]  FilterOutMin=[]  FilterOutMax=[]  SumI1OutMin=[]  SumI1OutMax=[]  SumI2OutMin=[]  SumI2OutMax=[]  SumI3OutMin=[]  SumI3OutMax=[]  SumI4OutMin=[]  SumI4OutMax=[]  SumDOutMin=[]  SumDOutMax=[]  DifferentiatorOutMin=[]  DifferentiatorOutMax=[]  FilterDiffOutCoefMin=[]  FilterDiffOutCoefMax=[]  ReciprocalOutMin=[]  ReciprocalOutMax=[]  SumDenOutMin=[]  SumDenOutMax=[]  SumNumOutMin=[]  SumNumOutMax=[]  DivideOutMin=[]  DivideOutMax=[]  UdiffTsProdOutMin=[]  UdiffTsProdOutMax=[]  NTsProdOutMin=[]  NTsProdOutMax=[]  UintegralTsProdOutMin=[]  UintegralTsProdOutMax=[]  UngainTsProdOutMin=[]  UngainTsProdOutMax=[]  ClampingZeroOutDataTypeStr=Inherit: Inherit via back propagation  ClampingZeroOutMin=[]  ClampingZeroOutMax=[]  FilterDenConstantOutDataTypeStr=Inherit: Inherit via back propagation  FilterDenConstantOutMin=[]  FilterDenConstantOutMax=[]  PCopyOutDataTypeStr=Inherit: Inherit via back propagation  PCopyOutMin=[]  PCopyOutMax=[]  NCopyOutDataTypeStr=Inherit: Inherit via back propagation  NCopyOutMin=[]  NCopyOutMax=[]  IntegratorContinuousStateAttributes=''  IntegratorStateMustResolveToSignalObject=off  IntegratorRTWStateStorageClass=Auto  FilterContinuousStateAttributes=''  FilterStateMustResolveToSignalObject=off  FilterRTWStateStorageClass=Auto  ParallelPVariant=InternalParameters  IdealPVariant=Disabled  IVariant=InternalParameters  DVariant=Disabled  IntegratorVariant=Discrete  SatVariant=Disabled  AWVariant=Passthrough  PCopyVariant=Disabled  TRVariant=Disabled  FdbkBlocksVariant=Forward  IdealPFdbkVariant=Disabled  SatFdbkVariant=Disabled  DerivativeFilterVariant=Disabled  NVariant=Disabled  NCopyVariant=Disabled_SignalSpec  FilterICVariant=Disabled  IntegratorICVariant=InternalICs  ExternalResetVariant=Disabled  TRSumVariant=Passthrough  SumFdbkVariant=Disabled  SumVariant=Sum_PI  TsampFilterVariant=InternalTs  TsampNgainVariant=Passthrough  TsampIntegralVariant=Disabled_SignalSpec  ExternalSaturationOutDataTypeStr=Inherit: Same as second input  DerivativeSourceVariant=Disabled  PreIntVariant=InternalPreInt
  PID Controller1 : slpidlib/PID Controller  Controller=PI  Form=Parallel  TimeDomain=Discrete-time  UseExternalTs=off  SampleTime=-1  IntegratorMethod=Forward Euler  FilterMethod=Forward Euler  ControllerParametersSource=internal  P=0.1  I=10000/200  UseKiTs=off  D=0  UseExternalDerivativeSource=off  N=100  UseFilter=on  TunerSelectOption=Transfer Function Based (PID Tuner App)  InitialConditionSource=internal  InitialConditionForIntegrator=0  InitialConditionForFilter=0  DifferentiatorICPrevScaledInput=0  ExternalReset=none  TrackingMode=off  Kt=1  LimitOutput=on  SatLimitsSource=internal  UpperSaturationLimit=20e3  LowerSaturationLimit=-20e3  LinearizeAsGain=on  AntiWindupMode=none  Kb=1  LimitIntegrator=off  UpperIntegratorSaturationLimit=inf  LowerIntegratorSaturationLimit=-inf  POutMin=[]  POutMax=[]  IOutMin=[]  IOutMax=[]  DOutMin=[]  DOutMax=[]  NOutMin=[]  NOutMax=[]  SumOutMin=[]  SumOutMax=[]  SaturationOutMin=[]  SaturationOutMax=[]  PParamMin=[]  PParamMax=[]  IParamMin=[]  IParamMax=[]  DParamMin=[]  DParamMax=[]  NParamMin=[]  NParamMax=[]  KbParamMin=[]  KbParamMax=[]  KtParamMin=[]  KtParamMax=[]  KbOutMin=[]  KbOutMax=[]  KtOutMin=[]  KtOutMax=[]  IntegratorOutMin=[]  IntegratorOutMax=[]  FilterOutMin=[]  FilterOutMax=[]  SumI1OutMin=[]  SumI1OutMax=[]  SumI2OutMin=[]  SumI2OutMax=[]  SumI3OutMin=[]  SumI3OutMax=[]  SumI4OutMin=[]  SumI4OutMax=[]  SumDOutMin=[]  SumDOutMax=[]  DifferentiatorOutMin=[]  DifferentiatorOutMax=[]  FilterDiffOutCoefMin=[]  FilterDiffOutCoefMax=[]  ReciprocalOutMin=[]  ReciprocalOutMax=[]  SumDenOutMin=[]  SumDenOutMax=[]  SumNumOutMin=[]  SumNumOutMax=[]  DivideOutMin=[]  DivideOutMax=[]  UdiffTsProdOutMin=[]  UdiffTsProdOutMax=[]  NTsProdOutMin=[]  NTsProdOutMax=[]  UintegralTsProdOutMin=[]  UintegralTsProdOutMax=[]  UngainTsProdOutMin=[]  UngainTsProdOutMax=[]  ClampingZeroOutDataTypeStr=Inherit: Inherit via back propagation  ClampingZeroOutMin=[]  ClampingZeroOutMax=[]  FilterDenConstantOutDataTypeStr=Inherit: Inherit via back propagation  FilterDenConstantOutMin=[]  FilterDenConstantOutMax=[]  PCopyOutDataTypeStr=Inherit: Inherit via back propagation  PCopyOutMin=[]  PCopyOutMax=[]  NCopyOutDataTypeStr=Inherit: Inherit via back propagation  NCopyOutMin=[]  NCopyOutMax=[]  IntegratorContinuousStateAttributes=''  IntegratorStateMustResolveToSignalObject=off  IntegratorRTWStateStorageClass=Auto  FilterContinuousStateAttributes=''  FilterStateMustResolveToSignalObject=off  FilterRTWStateStorageClass=Auto  ParallelPVariant=InternalParameters  IdealPVariant=Disabled  IVariant=InternalParameters  DVariant=Disabled  IntegratorVariant=Discrete  SatVariant=Enabled  AWVariant=Passthrough  PCopyVariant=Disabled  TRVariant=Disabled  FdbkBlocksVariant=Forward  IdealPFdbkVariant=Disabled  SatFdbkVariant=Disabled  DerivativeFilterVariant=Disabled  NVariant=Disabled  NCopyVariant=Disabled_SignalSpec  FilterICVariant=Disabled  IntegratorICVariant=InternalICs  ExternalResetVariant=Disabled  TRSumVariant=Passthrough  SumFdbkVariant=Disabled  SumVariant=Sum_PI  TsampFilterVariant=InternalTs  TsampNgainVariant=Passthrough  TsampIntegralVariant=Disabled_SignalSpec  ExternalSaturationOutDataTypeStr=Inherit: Same as second input  DerivativeSourceVariant=Disabled  PreIntVariant=InternalPreInt
  PID Controller2 : slpidlib/PID Controller  Controller=PI  Form=Parallel  TimeDomain=Discrete-time  UseExternalTs=off  SampleTime=-1  IntegratorMethod=Forward Euler  FilterMethod=Forward Euler  ControllerParametersSource=internal  P=0.1  I=1000/2  UseKiTs=off  D=0  UseExternalDerivativeSource=off  N=100  UseFilter=on  TunerSelectOption=Transfer Function Based (PID Tuner App)  InitialConditionSource=internal  InitialConditionForIntegrator=0  InitialConditionForFilter=0  DifferentiatorICPrevScaledInput=0  ExternalReset=none  TrackingMode=off  Kt=1  LimitOutput=on  SatLimitsSource=internal  UpperSaturationLimit=20e3  LowerSaturationLimit=-20e3  LinearizeAsGain=on  AntiWindupMode=none  Kb=1  LimitIntegrator=off  UpperIntegratorSaturationLimit=inf  LowerIntegratorSaturationLimit=-inf  POutMin=[]  POutMax=[]  IOutMin=[]  IOutMax=[]  DOutMin=[]  DOutMax=[]  NOutMin=[]  NOutMax=[]  SumOutMin=[]  SumOutMax=[]  SaturationOutMin=[]  SaturationOutMax=[]  PParamMin=[]  PParamMax=[]  IParamMin=[]  IParamMax=[]  DParamMin=[]  DParamMax=[]  NParamMin=[]  NParamMax=[]  KbParamMin=[]  KbParamMax=[]  KtParamMin=[]  KtParamMax=[]  KbOutMin=[]  KbOutMax=[]  KtOutMin=[]  KtOutMax=[]  IntegratorOutMin=[]  IntegratorOutMax=[]  FilterOutMin=[]  FilterOutMax=[]  SumI1OutMin=[]  SumI1OutMax=[]  SumI2OutMin=[]  SumI2OutMax=[]  SumI3OutMin=[]  SumI3OutMax=[]  SumI4OutMin=[]  SumI4OutMax=[]  SumDOutMin=[]  SumDOutMax=[]  DifferentiatorOutMin=[]  DifferentiatorOutMax=[]  FilterDiffOutCoefMin=[]  FilterDiffOutCoefMax=[]  ReciprocalOutMin=[]  ReciprocalOutMax=[]  SumDenOutMin=[]  SumDenOutMax=[]  SumNumOutMin=[]  SumNumOutMax=[]  DivideOutMin=[]  DivideOutMax=[]  UdiffTsProdOutMin=[]  UdiffTsProdOutMax=[]  NTsProdOutMin=[]  NTsProdOutMax=[]  UintegralTsProdOutMin=[]  UintegralTsProdOutMax=[]  UngainTsProdOutMin=[]  UngainTsProdOutMax=[]  ClampingZeroOutDataTypeStr=Inherit: Inherit via back propagation  ClampingZeroOutMin=[]  ClampingZeroOutMax=[]  FilterDenConstantOutDataTypeStr=Inherit: Inherit via back propagation  FilterDenConstantOutMin=[]  FilterDenConstantOutMax=[]  PCopyOutDataTypeStr=Inherit: Inherit via back propagation  PCopyOutMin=[]  PCopyOutMax=[]  NCopyOutDataTypeStr=Inherit: Inherit via back propagation  NCopyOutMin=[]  NCopyOutMax=[]  IntegratorContinuousStateAttributes=''  IntegratorStateMustResolveToSignalObject=off  IntegratorRTWStateStorageClass=Auto  FilterContinuousStateAttributes=''  FilterStateMustResolveToSignalObject=off  FilterRTWStateStorageClass=Auto  ParallelPVariant=InternalParameters  IdealPVariant=Disabled  IVariant=InternalParameters  DVariant=Disabled  IntegratorVariant=Discrete  SatVariant=Enabled  AWVariant=Passthrough  PCopyVariant=Disabled  TRVariant=Disabled  FdbkBlocksVariant=Forward  IdealPFdbkVariant=Disabled  SatFdbkVariant=Disabled  DerivativeFilterVariant=Disabled  NVariant=Disabled  NCopyVariant=Disabled_SignalSpec  FilterICVariant=Disabled  IntegratorICVariant=InternalICs  ExternalResetVariant=Disabled  TRSumVariant=Passthrough  SumFdbkVariant=Disabled  SumVariant=Sum_PI  TsampFilterVariant=InternalTs  TsampNgainVariant=Passthrough  TsampIntegralVariant=Disabled_SignalSpec  ExternalSaturationOutDataTypeStr=Inherit: Same as second input  DerivativeSourceVariant=Disabled  PreIntVariant=InternalPreInt
  Saturation : Saturate  UpperLimit=1  LowerLimit=-1
  Scope : Scope  NumInputPorts=2
  Scope4 : Scope  NumInputPorts=2
  Sum : Sum  Inputs=|-+
  Sum1 : Sum  Inputs=|+-
  Sum2 : Sum  Inputs=|+-
  Sum3 : Sum  Inputs=|+-
  Sum{4..6,8} (4 alike) : Sum  Inputs=|++
  Switch : Switch  Criteria=u2 > Threshold  Threshold=10
  Terminator : Terminator
  Terminator1 : Terminator
  abc to dq0 : spsabctodq0Lib/abc to dq0  Alignment=90 degrees behind phase A axis
  abc to dq1 : spsabctodq0Lib/abc to dq0  Alignment=90 degrees behind phase A axis
  dq0 to abc : spsdq0toabcLib/dq0 to abc  Alignment=90 degrees behind phase A axis
  wL : Gain  Gain=0.314*0.003
  wL1 : Gain  Gain=0.314*0.003
  Pulses : Outport
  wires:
  abc to dq0/1 -> Demux/1
  Demux/3 -> Terminator/1
  Demux1/3 -> Terminator1/1
  abc to dq1/1 -> Demux1/1
  Iabc_B3/1 -> abc to dq1/1
  Constant/1 -> Sum/1
  Demux/2 -> [Vq]  "Vq"
  Sum/1 -> PID Controller/1
  PID Controller/1 -> Sum8/1
  [wt] -> abc to dq1/2, abc to dq0/2
  Demux1/1 -> [Id]  "Id"
  Demux1/2 -> [Iq]  "Iq"
  [Id] -> Scope/2, Sum1/2
  Iqref/1 -> Scope4/1, Sum2/1
  [Iq] -> Sum2/2, Scope4/2
  Sum1/1 -> PID Controller1/1
  Sum2/1 -> PID Controller2/1
  PID Controller1/1 -> Sum3/1
  PID Controller2/1 -> Sum4/1
  wL1/1 -> Sum4/2
  wL/1 -> Sum3/2
  Sum3/1 -> Sum5/1
  [Vd] -> Sum5/2
  Sum4/1 -> Sum6/1
  [Vq] -> Sum6/2
  Mux/1 -> dq0 to abc/1
  Sum5/1 -> Mux/1  "ud"
  Sum6/1 -> Mux/2  "uq"
  Constant1/1 -> Mux/3
  dq0 to abc/1 -> Gain/1
  Vabc_B3/1 -> abc to dq0/1
  Idref/1 -> Scope/1, Sum1/1
  [Id] -> wL1/1
  [Iq] -> wL/1
  Demux/1 -> [Vd]  "Vd"
  Gain/1 -> Saturation/1
  Memory/1 -> Pulses/1
  Discrete-Time Integrator/1 -> [wt]
  Saturation/1 -> Memory/1
  Constant3/1 -> Sum8/2
  Switch/1 -> Sum/2
  Constant4/1 -> Switch/3
  Clock/1 -> Switch/2
  [Vq] -> Switch/1
  [wt] -> dq0 to abc/2
  Sum8/1 -> Discrete-Time Integrator/1
